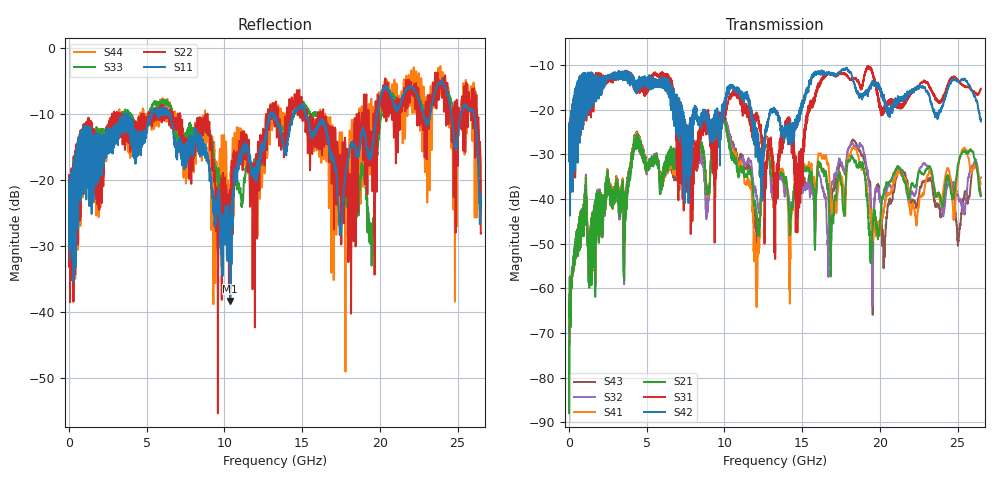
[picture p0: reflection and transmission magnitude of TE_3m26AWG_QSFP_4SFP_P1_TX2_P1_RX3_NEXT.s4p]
!Agilent Technologies,N5222A,MY51421691,A.10.00.00
!Agilent N5222A: A.10.00.00
!Date: Friday, January 30, 2015 12:34:32
!Correction: S11(Full 4 Port(1,2,3,4))
!S12(Full 4 Port(1,2,3,4))
!S13(Full 4 Port(1,2,3,4))
!S14(Full 4 Port(1,2,3,4))
!S21(Full 4 Port(1,2,3,4))
!S22(Full 4 Port(1,2,3,4))
!S23(Full 4 Port(1,2,3,4))
!S24(Full 4 Port(1,2,3,4))
!S31(Full 4 Port(1,2,3,4))
!S32(Full 4 Port(1,2,3,4))
!S33(Full 4 Port(1,2,3,4))
!S34(Full 4 Port(1,2,3,4))
!S41(Full 4 Port(1,2,3,4))
!S42(Full 4 Port(1,2,3,4))
!S43(Full 4 Port(1,2,3,4))
!S44(Full 4 Port(1,2,3,4))
!S4P File: Measurements: <S11,S12,S13,S14>,
!<S21,S22,S23,S24>,
!<S31,S32,S33,S34>,
!<S41,S42,S43,S44>:
# Hz S  dB  R 50.0
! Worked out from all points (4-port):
!   2650 points, 10 MHz to 26.5 GHz, reference 50 ohm
!   strongest paths, dB at 10 MHz, 6.63 GHz, 13.26 GHz, 19.88 GHz, 26.5 GHz:
!     S42: -25.0, -15.7, -19.8, -13.9, -22.6
!     S31: -24.7, -15.5, -42.3, -17.3, -15.3
!     S21: -71.8, -28.8, -34.8, -49.0, -39.3
!     S41: -70.2, -29.3, -34.7, -46.1, -36.6
!     S32: -67.7, -29.3, -37.1, -37.8, -35.2
!     S43: -64.1, -29.7, -36.4, -36.6, -39.3
!   lowest |S11| = -38.4 dB at 10.38 GHz (marker M1), VSWR 1.02, Z = 49.1 + j0.742 ohm
!   |S11| at or under -10 dB: start of sweep to 3.58 GHz; 6.485 GHz to 12.98 GHz (6.493 GHz wide, 66.7 % of centre); 15.24 GHz to 19.8 GHz (4.557 GHz wide, 26 % of centre)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
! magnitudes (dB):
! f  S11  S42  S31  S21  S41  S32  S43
! 10 MHz  -19.9  -25.0  -24.7  -71.8  -70.2  -67.7  -64.1
! 4.3 GHz  -13.1  -13.8  -14.2  -26.6  -26.3  -26.2  -26.0
! 10.38 GHz  -38.4  -15.0  -17.6  -29.1  -28.7  -26.7  -26.3
! 12.04 GHz  -18.0  -26.6  -21.8  -43.4  -60.6  -39.3  -48.2
! 12.69 GHz  -13.2  -23.4  -32.5  -28.0  -26.3  -28.1  -26.0
! 14.23 GHz  -11.6  -25.3  -22.3  -46.8  -51.5  -42.3  -44.7
! 26.5 GHz  -22.2  -22.6  -15.3  -39.3  -36.6  -35.2  -39.3
